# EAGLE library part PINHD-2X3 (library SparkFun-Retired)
PIN HEADER
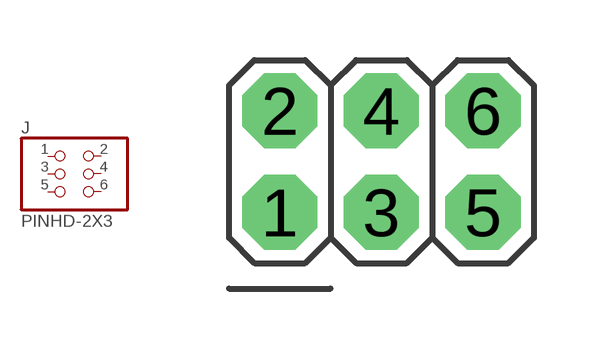
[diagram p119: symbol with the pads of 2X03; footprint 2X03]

Designator prefix J

## PINHD-2X3  [2X03]
1  1  pas
2  2  pas
3  3  pas
4  4  pas
5  5  pas
6  6  pas

## Footprint 2X03 (pad centres in mm)
PIN HEADER
drill 1.016 pad 1.88 octagon: 1 -2.54,-1.27; 2 -2.54,1.27; 3 0,-1.27; 4 0,1.27; 5 2.54,-1.27; 6 2.54,1.27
